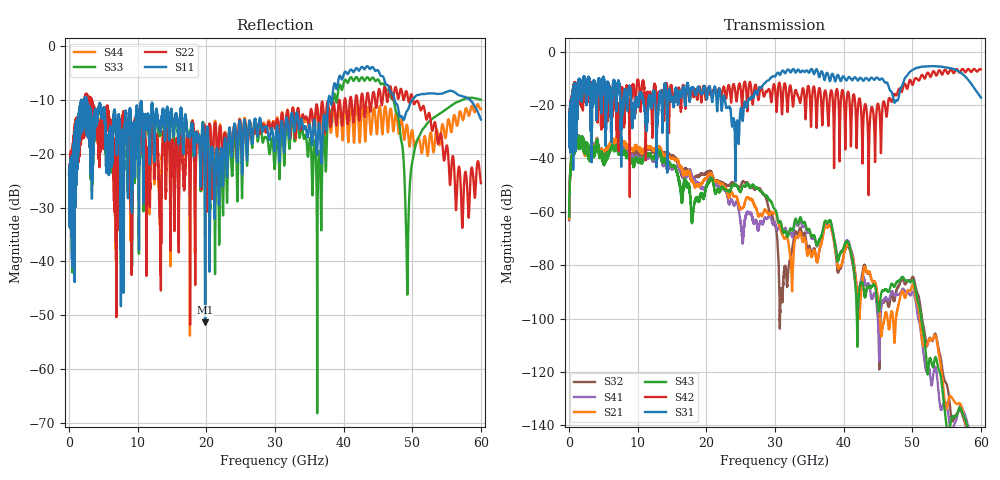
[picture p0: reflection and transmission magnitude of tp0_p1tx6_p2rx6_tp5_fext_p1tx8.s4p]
! 100G CR Analysis
! File: tp0_p1tx6_p2rx6_tp5_fext_p1tx8
! Description: 2m Cu Cable, OSFP, TP0-TP5
! Port Mapping
! Port1 -- P1TX8N
! Port2 -- P2RX6N
! Port3 -- P1TX8P
! Port4 -- P2RX6P
# GHz S MA R 50.00
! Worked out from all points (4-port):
!   6000 points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, 10 MHz to 60 GHz, reference 50 ohm
!   strongest paths, dB at 10 MHz, 15.01 GHz, 30.01 GHz, 45.01 GHz, 60 GHz:
!     S31: -28.1, -17.8, -9.3, -10.0, -17.2
!     S42: -27.9, -14.2, -13.6, -19.5, -6.7
!     S43: -61.9, -43.2, -59.2, -95.9, -153.2
!     S21: -62.6, -40.0, -60.3, -92.3, -147.1
!     S41: -61.4, -44.1, -63.9, -101.2, -149.1
!     S32: -63.1, -39.1, -65.2, -97.4, -149.8
!   lowest |S11| = -51.3 dB at 19.82 GHz (marker M1), VSWR 1.01, Z = 50.2 + j0.113 ohm
!   |S11| at or under -10 dB: start of sweep to 1.808 GHz; 2.56 GHz to 37.79 GHz (35.23 GHz wide, 175 % of centre); 47.43 GHz to 49.99 GHz (2.559 GHz wide, 5.25 % of centre)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
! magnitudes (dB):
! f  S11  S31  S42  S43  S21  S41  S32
! 10 MHz  -23.8  -28.1  -27.9  -61.9  -62.6  -61.4  -63.1
! 1.34 GHz  -14.8  -16.6  -19.0  -31.5  -31.6  -31.3  -31.3
! 19.82 GHz  -51.3  -13.3  -16.2  -53.0  -47.9  -51.3  -46.1
! 30.85 GHz  -15.0  -8.2  -15.1  -63.9  -67.0  -65.6  -88.9
! 45.06 GHz  -4.6  -10.1  -19.7  -96.7  -93.2  -103.5  -100.1
! 49.27 GHz  -12.0  -8.9  -13.9  -85.6  -89.7  -90.2  -85.8
! 60 GHz  -13.6  -17.2  -6.7  -153.2  -147.1  -149.1  -149.8
